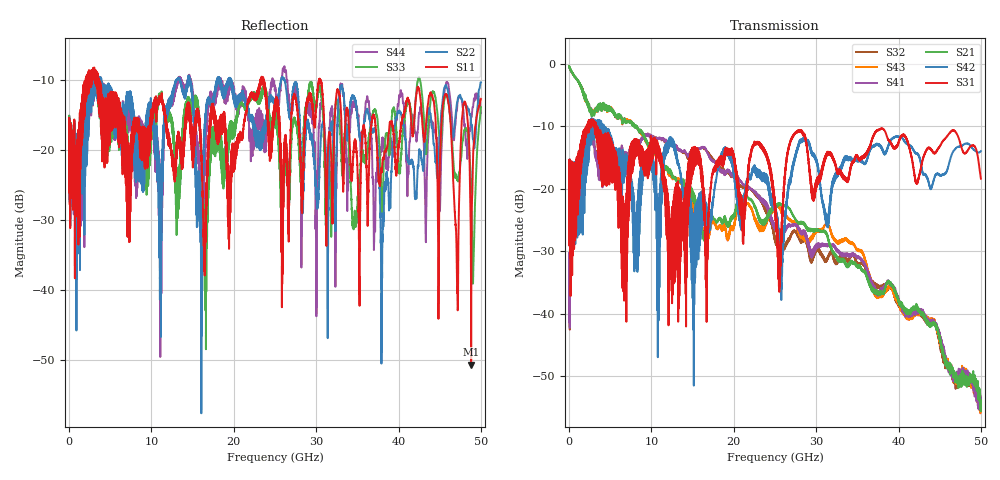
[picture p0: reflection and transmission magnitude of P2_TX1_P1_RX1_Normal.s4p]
!Keysight Technologies,N5225A,MY51441389,A.10.49.11
!Date: Monday, July 08, 2019 13:14:36
!Correction: S11(Full 4 Port(1,2,3,4))
!S12(Full 4 Port(1,2,3,4))
!S13(Full 4 Port(1,2,3,4))
!S14(Full 4 Port(1,2,3,4))
!S21(Full 4 Port(1,2,3,4))
!S22(Full 4 Port(1,2,3,4))
!S23(Full 4 Port(1,2,3,4))
!S24(Full 4 Port(1,2,3,4))
!S31(Full 4 Port(1,2,3,4))
!S32(Full 4 Port(1,2,3,4))
!S33(Full 4 Port(1,2,3,4))
!S34(Full 4 Port(1,2,3,4))
!S41(Full 4 Port(1,2,3,4))
!S42(Full 4 Port(1,2,3,4))
!S43(Full 4 Port(1,2,3,4))
!S44(Full 4 Port(1,2,3,4))
!S4P File: Measurements: <S11,S12,S13,S14>,
!<S21,S22,S23,S24>,
!<S31,S32,S33,S34>,
!<S41,S42,S43,S44>:
# Hz S  dB  R 50
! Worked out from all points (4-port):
!   5000 points, 10 MHz to 50 GHz, reference 50 ohm
!   strongest paths, dB at 10 MHz, 12.51 GHz, 25.01 GHz, 37.51 GHz, 50 GHz:
!     S31: -19.0, -38.3, -22.9, -10.6, -18.4
!     S42: -19.0, -12.6, -23.2, -12.8, -14.0
!     S21: -0.4, -17.7, -22.7, -36.7, -55.6
!     S41: -33.0, -12.6, -26.5, -36.9, -54.0
!     S43: -0.4, -18.1, -22.9, -37.2, -53.8
!     S32: -32.9, -13.0, -28.5, -35.7, -55.5
!   lowest |S11| = -50.7 dB at 48.82 GHz (marker M1), VSWR 1.01, Z = 50.2 + j0.211 ohm
!   |S11| at or under -10 dB: 3.66 GHz to 23.22 GHz (19.56 GHz wide, 146 % of centre); 23.67 GHz to 30.34 GHz (6.672 GHz wide, 24.7 % of centre); 30.55 GHz to end of sweep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
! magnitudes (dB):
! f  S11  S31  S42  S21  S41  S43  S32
! 10 MHz  -17.8  -19.0  -19.0  -0.4  -33.0  -0.4  -32.9
! 2.07 GHz  -10.2  -10.5  -12.4  -6.1  -11.4  -6.1  -11.3
! 16.29 GHz  -29.6  -22.1  -24.9  -27.9  -13.3  -27.3  -13.4
! 23.42 GHz  -9.5  -13.5  -17.9  -25.3  -22.2  -26.3  -22.4
! 25.51 GHz  -17.2  -30.3  -28.1  -22.4  -27.2  -23.0  -29.6
! 48.82 GHz  -50.7  -13.2  -13.3  -50.2  -50.6  -51.8  -51.0
! 50 GHz  -12.7  -18.4  -14.0  -55.6  -54.0  -53.8  -55.5
